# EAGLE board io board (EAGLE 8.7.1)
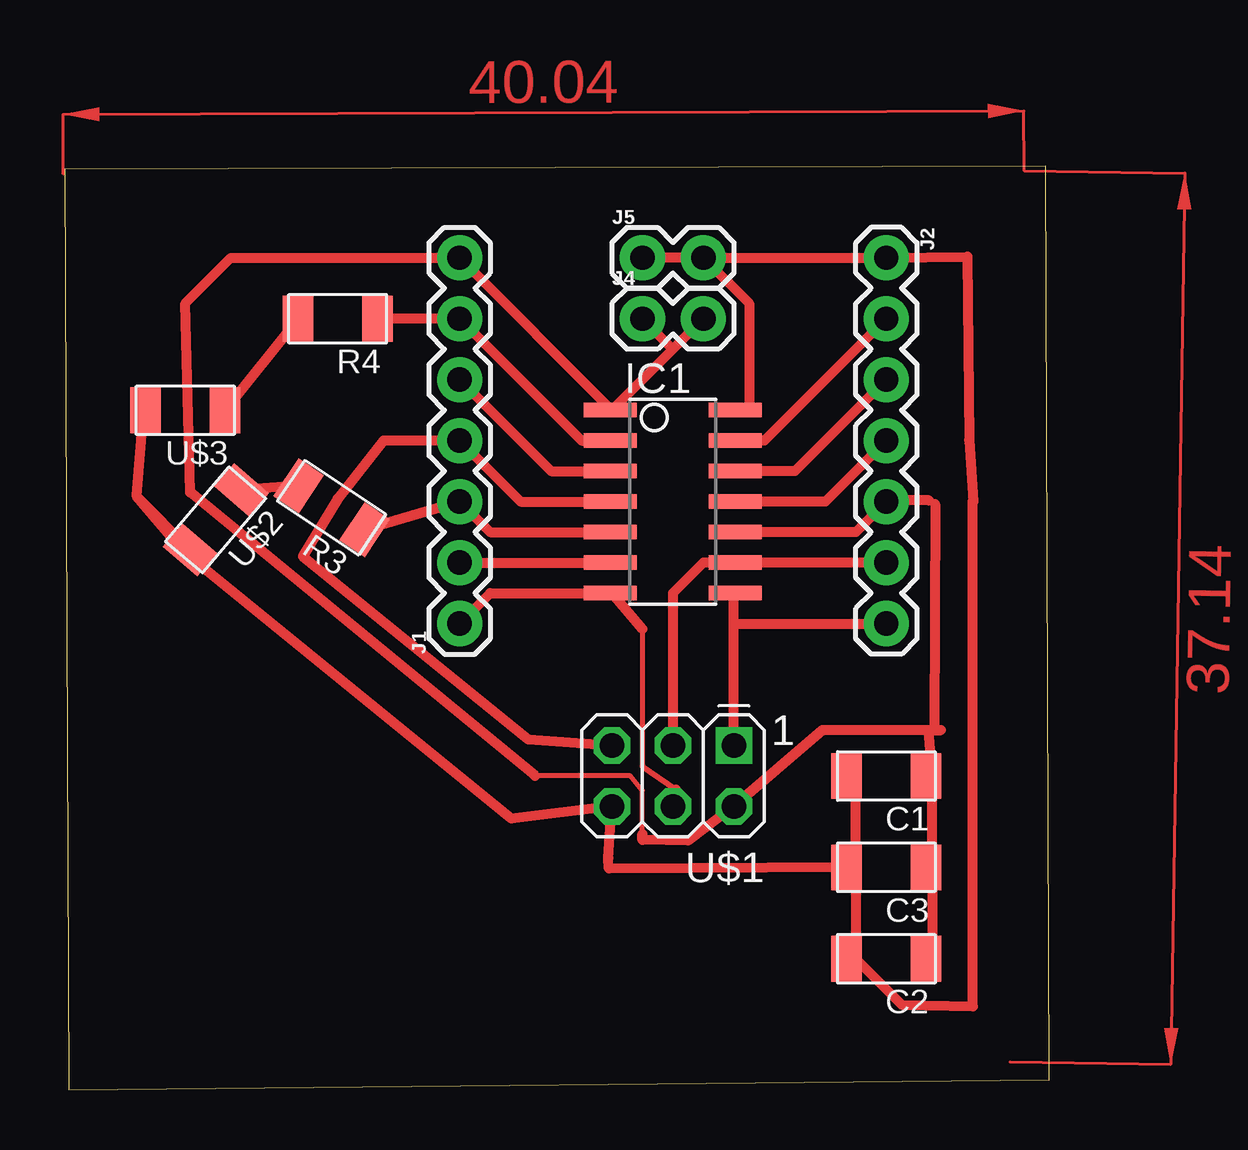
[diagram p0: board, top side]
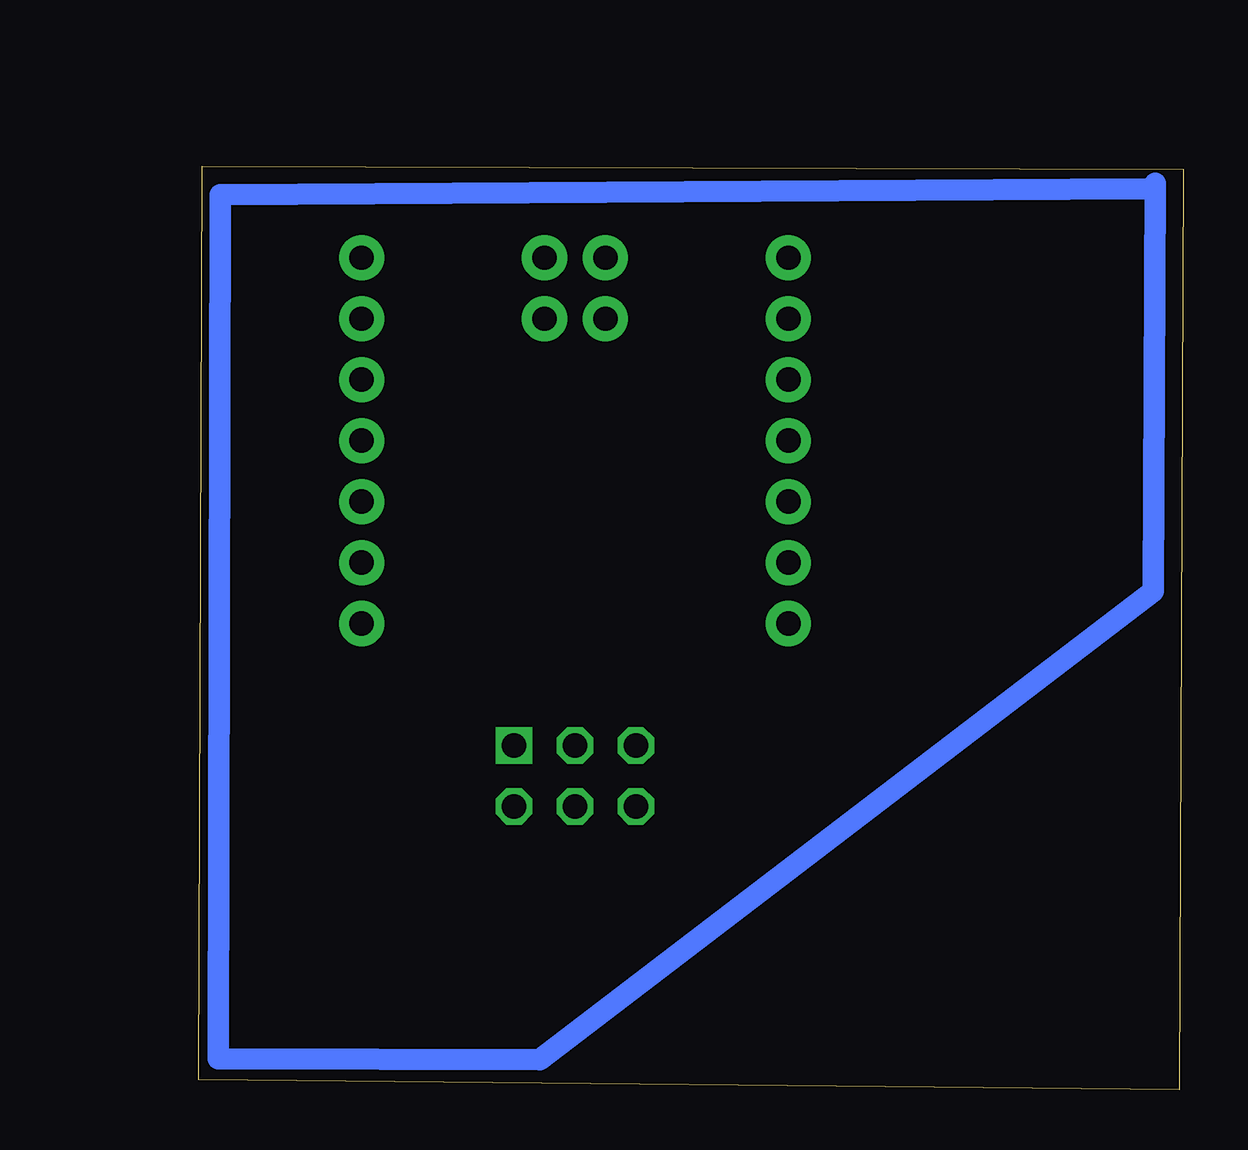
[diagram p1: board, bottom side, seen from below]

Size 41.03 x 38.48 mm. Coordinates in mm from the lower left corner, seen from the top.
Outline: 0.18,0 41.03,0.43 40.87,38.48 0,38.35 0.18,0
Copper layers (1*16): Top 0.035mm / dielectric 1.5mm / Bottom 0.035mm
Design rules "default *": minimum track width 16mil, minimum drill 0.35mm, track to track 16mil, track to pad 16mil, pad to pad 16mil, via to via 16mil, smd to smd 16mil, copper to edge 40mil, drill to drill 6mil, minimum pad ring 10mil, minimum via ring 8mil, stop-mask expansion 4mil, vias tented up to drill 0mil, thermal gap 10mil

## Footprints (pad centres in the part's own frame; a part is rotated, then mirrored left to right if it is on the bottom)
C1206FAB = smd 1.27 x 1.905: 1 -1.651,0; 2 1.651,0
SOIC14 = smd 0.61 x 2.21: 1 -3.81,-2.603; 2 -2.54,-2.603; 3 -1.27,-2.603; 4 0,-2.603; 5 1.27,-2.603; 6 2.54,-2.603; 7 3.81,-2.603; 8 3.81,2.603; 9 2.54,2.603; 10 1.27,2.603; 11 0,2.603; 12 -1.27,2.603; 13 -2.54,2.603; 14 -3.81,2.603
1X07 = drill 1.016 pad 1.88: 1 0,0; 2 2.54,0; 3 5.08,0; 4 7.62,0; 5 10.16,0; 6 12.7,0; 7 15.24,0
1X02 = drill 1.016 pad 1.88: 1 0,0; 2 2.54,0
R1206FAB = smd 1.27 x 1.905: 1 -1.651,0; 2 1.651,0
2X03 = drill 1.016 square: 1 -2.54,-1.27 | drill 1.016 octagon: 2 -2.54,1.27; 3 0,-1.27; 4 0,1.27; 5 2.54,-1.27; 6 2.54,1.27
LED1206FAB = smd 1.27 x 1.905: 1 -1.651,0; 2 1.651,0

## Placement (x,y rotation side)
C1  100nf  [C1206FAB]  34.24,13.08 180 top
C2  1uf  [C1206FAB]  34.24,5.46 180 top
C3  10uf  [C1206FAB]  34.24,9.27 180 top
IC1  ATTINY44-SSU  [SOIC14]  25.35,24.51 270 top
J1  [1X07]  16.46,19.43 90 top
J2  [1X07]  34.24,34.67 270 top
J4  [1X02]  24.08,32.13 0 top
J5  [1X02]  24.08,34.67 0 top
R3  499  [R1206FAB]  11.13,24.26 146.3 top
R4  499  [R1206FAB]  11.38,32.13 180 top
U$1  AVRISP  [2X03]  25.35,13.08 180 top
U$2  LEDFAB1206  [LED1206FAB]  6.3,23.75 229.4 top
U$3  LEDFAB1206  [LED1206FAB]  5.03,28.32 180 top

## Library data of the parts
C1-C3 IC1 R3 R4 U$1-U$3 = fab
J1 J2 J4 J5 = SparkFun-Connectors

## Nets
2: IC1.2 J1.6 R4.1
3: IC1.3 J1.5
4: IC1.4 J1.4 U$1.5
5: IC1.5 J1.3 R3.1
6: IC1.6 J1.2
7: IC1.7 J1.1 U$1.4
8: IC1.8 J2.7 U$1.1
9: IC1.9 J2.6 U$1.3
11: IC1.11 J2.4
12: IC1.12 J2.3
13: IC1.13 J2.2
GND: C1.2 C2.2 C3.2 IC1.14 J2.1 J5.1 J5.2 U$1.6 U$2.2 U$3.2
LED: R3.2 U$2.1
LED1: R4.2 U$3.1
S$1: IC1.10 J2.5
VCC: C1.1 C2.1 C3.1 IC1.1 J1.7 J4.1 J4.2 U$1.2

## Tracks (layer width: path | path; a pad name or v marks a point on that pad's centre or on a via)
2
  Top 0.406: R4.1 J1.6 21.54,27.05 IC1.2
3
  Top 0.406: IC1.3 20.27,25.78 J1.5
4
  Top 0.406: IC1.4 19,24.51 J1.4 13.28,27.05 11.38,24.64 9.93,22.23 19.33,14.61 U$1.5
5
  Top 0.406: R3.1 J1.3 17.73,23.24 IC1.5
6
  Top 0.406: J1.2 IC1.6
7
  Top 0.203: 24.08,19.2 24.08,13.49
  Top 0.254: 24.08,13.49 25.48,12.52
  Top 0.406: J1.1 17.73,20.7 IC1.7 22.81,20.7 24.08,19.2 | 25.48,12.52 U$1.4
8
  Top 0.406: U$1.1 27.89,19.43 | 27.89,19.43 27.89,20.7 IC1.8 | 27.89,19.43 J2.7
9
  Top 0.406: J2.6 IC1.9 26.62,21.97 25.35,20.7 U$1.3
10
  Top 0.406: 36.27,24.41 36.25,14.99
11
  Top 0.406: IC1.11 31.7,24.51 J2.4
12
  Top 0.406: IC1.12 30.43,25.78 J2.3
13
  Top 0.406: IC1.13 29.16,27.05 J2.2
GND
  Top 0.406: J5.2 28.52,32.77 28.52,28.32 IC1.14 | J5.2 J5.1 | J5.2 J2.1 37.62,34.72 37.69,27.08 37.87,24.51 37.85,24.56 37.85,3.48 34.87,3.56 32.97,5.46 | 3,24.77 3.25,28.07 U$3.2 | 32.97,9.27 32.97,5.46 | 32.97,9.27 32.97,13.08 C1.2 | 32.97,9.27 C3.2 22.68,9.22 22.66,9.65 U$1.6 18.62,11.3 5.03,22.35 3,24.77 | 3,24.77 U$2.2 | 32.97,5.46 C2.2
LED
  Top 0.406: R3.2 U$2.1
LED1
  Top 0.406: R4.2 U$3.1
N$2
  Bottom 0.889: 1.47,37.54 40.13,37.29 40.21,1.3 26.82,1.25 1.24,20.78 1.17,37.77
S$1
  Top 0.406: J2.5 32.97,23.24 IC1.10
S$2
  Top 0.406: 36.02,24.56 34.32,24.56
VCC
  Top 0.203: 19.61,13.08 23.57,13.08 24.08,12.47 24.08,10.67
  Top 0.406: 22.81,28.32 J4.2 25.35,30.86 J4.1 | 22.81,28.32 J1.7 6.93,34.67 5.03,32.77 5.23,24.89 19.61,13.08 | 22.81,28.32 IC1.1 | 36.14,9.27 36.14,5.46 C2.1 | 36.14,9.27 36.14,13.08 | 36.14,9.27 C3.1 | 36.14,13.08 36.02,14.99 | 36.02,14.99 36.53,14.99 | 36.14,13.08 C1.1 | 36.02,14.99 31.57,14.99 U$1.2 25.98,10.39 24.08,10.41 24.08,10.67
(copper drawn outside any net)
  shapes: Top area x2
